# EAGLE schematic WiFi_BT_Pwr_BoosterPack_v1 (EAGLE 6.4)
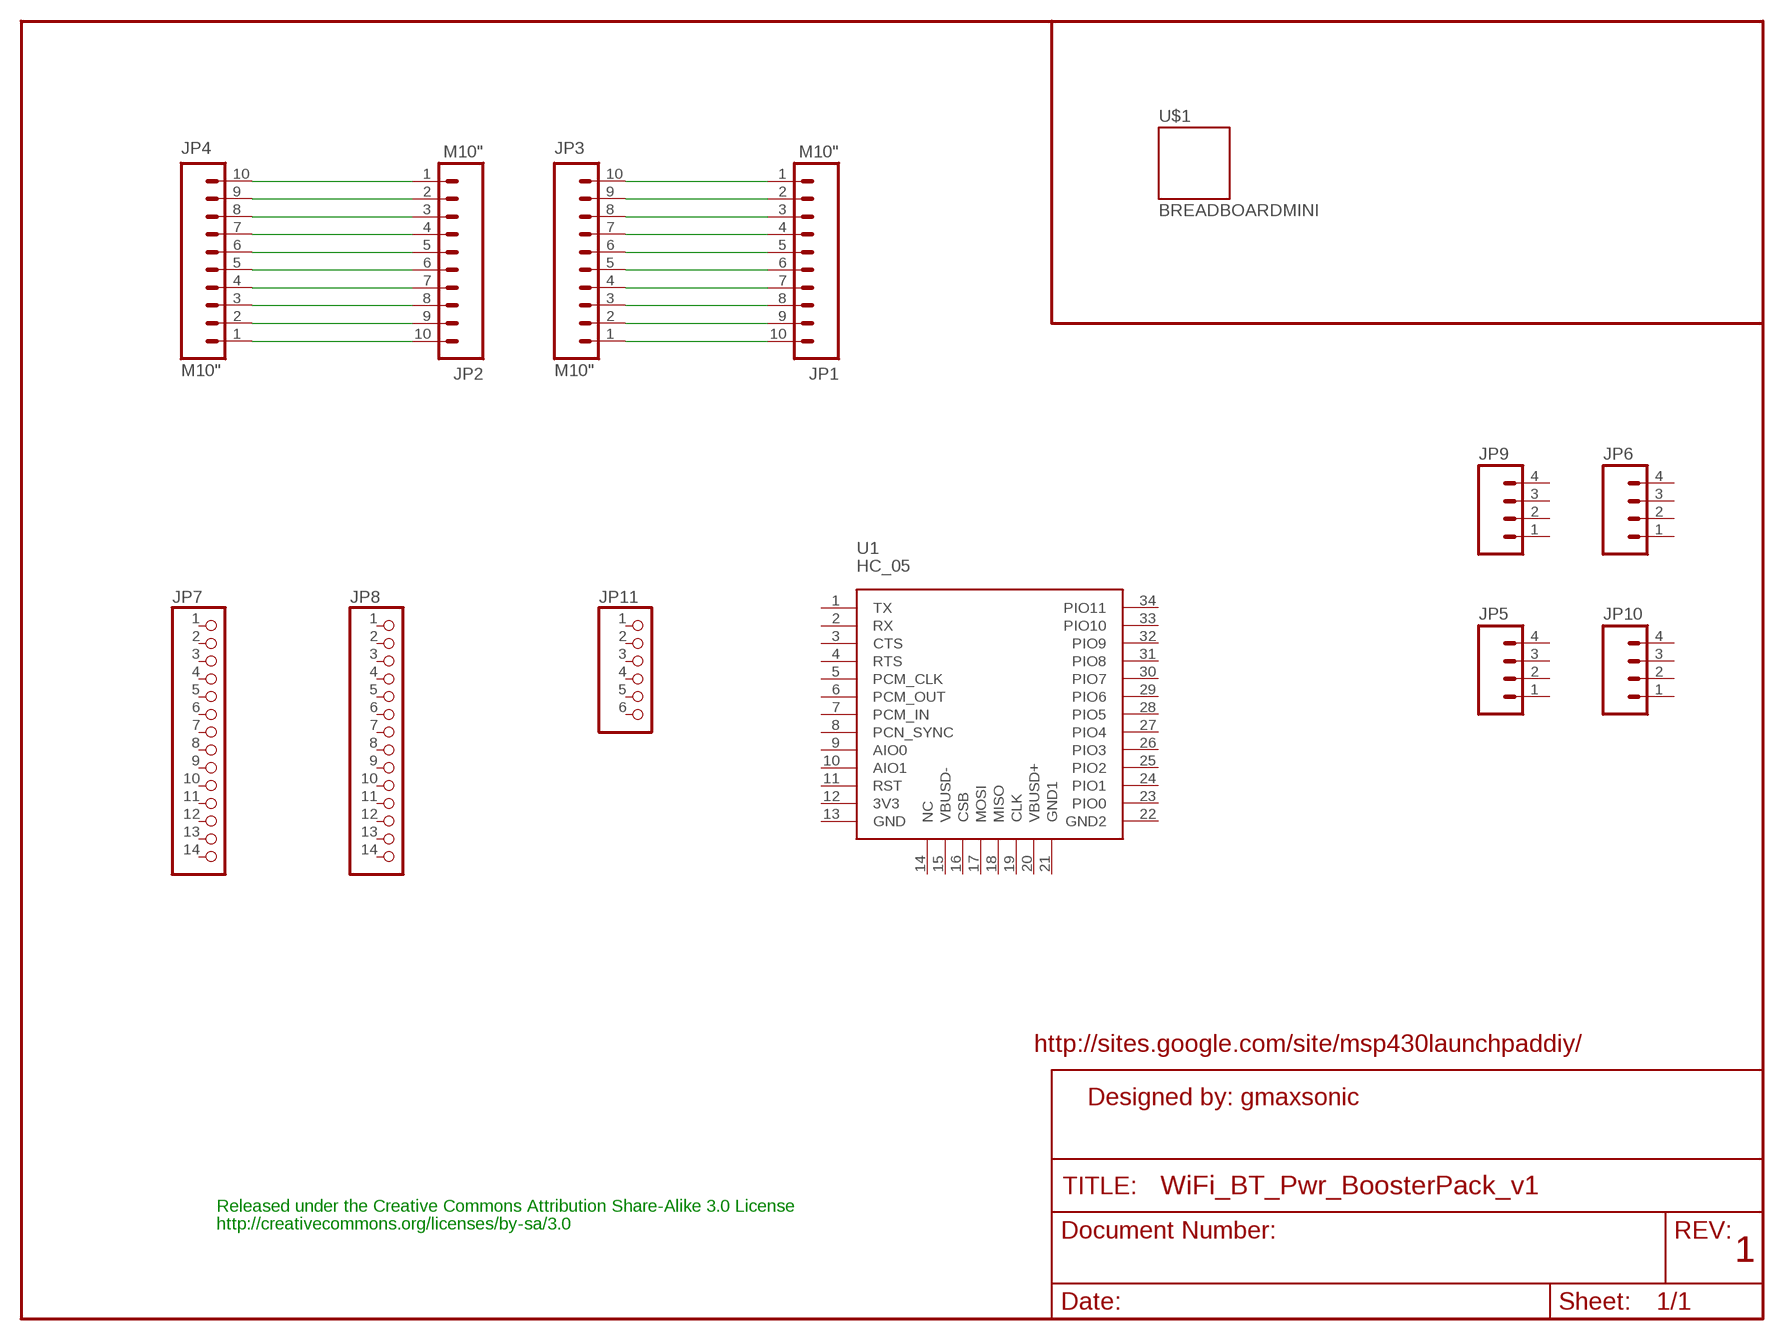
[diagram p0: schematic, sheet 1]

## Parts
JP1  M10"  [1X10]
JP2  M10"  [1X10]
JP3  M10"  [1X10]
JP4  M10"  [1X10]
JP5  M04PTH  [1X04]
JP6  M04PTH  [1X04]
JP7  PINHD-1X14M  [1X14M]
JP8  PINHD-1X14M  [1X14M]
JP9  M04PTH  [1X04]
JP10  M04PTH  [1X04]
JP11  PINHD-1X6  [1X06]
U1  HC_05  [BLUETOOTH_SMD]
U$1  BREADBOARDMINI  [BREADBOARD-MINI]

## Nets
N$1: JP2.1 JP4.10
N$2: JP2.2 JP4.9
N$3: JP2.3 JP4.8
N$4: JP2.4 JP4.7
N$5: JP2.5 JP4.6
N$6: JP2.6 JP4.5
N$7: JP2.7 JP4.4
N$8: JP2.8 JP4.3
N$9: JP2.9 JP4.2
N$10: JP2.10 JP4.1
N$11: JP1.1 JP3.10
N$12: JP1.2 JP3.9
N$13: JP1.3 JP3.8
N$14: JP1.4 JP3.7
N$15: JP1.5 JP3.6
N$16: JP1.6 JP3.5
N$17: JP1.7 JP3.4
N$18: JP1.8 JP3.3
N$19: JP1.9 JP3.2
N$20: JP1.10 JP3.1
Unconnected: JP5.1 JP5.2 JP5.3 JP5.4 JP6.1 JP6.2 JP6.3 JP6.4 JP7.1 JP7.2 JP7.3 JP7.4 JP7.5 JP7.6 JP7.7 JP7.8 JP7.9 JP7.10 JP7.11 JP7.12 JP7.13 JP7.14 JP8.1 JP8.2 JP8.3 JP8.4 JP8.5 JP8.6 JP8.7 JP8.8 JP8.9 JP8.10 JP8.11 JP8.12 JP8.13 JP8.14 JP9.1 JP9.2 JP9.3 JP9.4 JP10.1 JP10.2 JP10.3 JP10.4 JP11.1 JP11.2 JP11.3 JP11.4 JP11.5 JP11.6 U1.1(TX) U1.2(RX) U1.3(CTS) U1.4(RTS) U1.5(PCM_CLK) U1.6(PCM_OUT) U1.7(PCM_IN) U1.8(PCN_SYNC) U1.9(AIO0) U1.10(AIO1) U1.11(RST) U1.12(3V3) U1.13(GND) U1.14(NC) U1.15(VBUSD-) U1.16(CSB) U1.17(MOSI) U1.18(MISO) U1.19(CLK) U1.20(VBUSD+) U1.21(GND1) U1.22(GND2) U1.23(PIO0) U1.24(PIO1) U1.25(PIO2) U1.26(PIO3) U1.27(PIO4) U1.28(PIO5) U1.29(PIO6) U1.30(PIO7) U1.31(PIO8) U1.32(PIO9) U1.33(PIO10) U1.34(PIO11)

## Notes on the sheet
- http://sites.google.com/site/msp430launchpaddiy/
- Designed by: gmaxsonic
- Released under the Creative Commons Attribution Share-Alike 3.0 License
- http://creativecommons.org/licenses/by-sa/3.0
- 1

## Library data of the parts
JP1-JP4 = SparkFun:M10: Header 10 Standard 10-pin 0.1" header. Use with straight break away headers (SKU : PRT-00116), right angle break away headers (PRT-00553), swiss pins (PRT-00743), machine pins (PRT-00117), and female headers (PRT-00115).
JP5 JP6 JP9 JP10 = SparkFun:M04: Header 4 Standard 4-pin 0.1" header. Use with straight break away headers (SKU : PRT-00116), right angle break away headers (PRT-00553), swiss pins (PRT-00743), machine pins (PRT-00117), and female headers (PRT-00115). Molex polarized connector foot print use with SKU : PRT-08231 with associated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
JP7 JP8 = pinhead-2:PINHD-1X14: PIN HEADER
JP11 = pinhead-2:PINHD-1X6: PIN HEADER
U1 = SerialPortBluetooth:HC_05
U$1 = SparkFun:BREADBOARD: Breadboard Mini Self Adhesive

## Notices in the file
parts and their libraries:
SparkFun-Connectors: Licensing: CC v3.0 Share-Alike You are welcome to use this library for commercial purposes.
